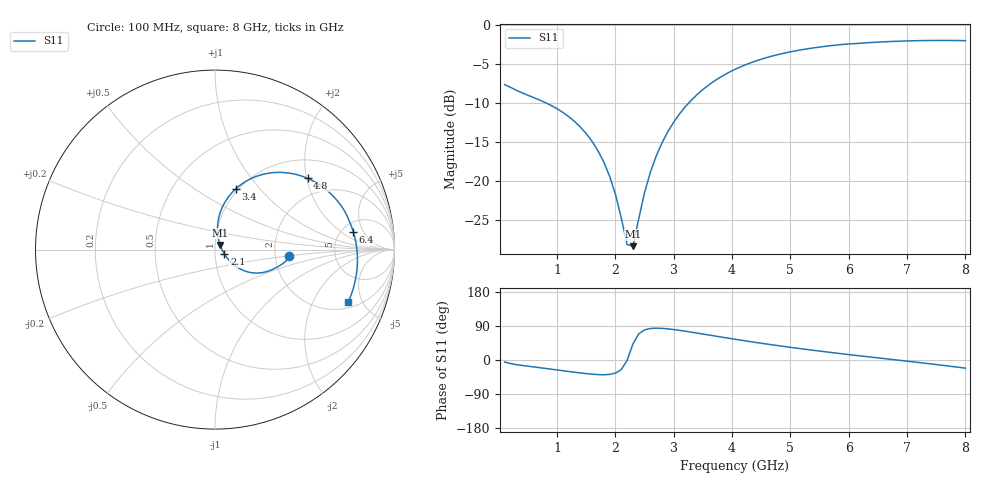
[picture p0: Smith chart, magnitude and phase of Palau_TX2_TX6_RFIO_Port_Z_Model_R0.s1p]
! Created Wed Jul  8 18:09:28 2020
! Palau TX2/TX6 RFIO Port Impedance Model.
! Revision		: R0.
! Impedance Mode 	: Balanced Differential-Mode.
! Impedance Format 	: Series Equivalent Differential Impedance (SEDZ).
# hz S ma R 50
! 1 Port Network Data from SP1.SP block
! freq  magS11  angS11
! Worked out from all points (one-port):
!   80 points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, 100 MHz to 8 GHz, reference 50 ohm
!   lowest |S11| = -28.4 dB at 2.3 GHz (marker M1), VSWR 1.08, Z = 52.8 + j2.7 ohm
!   |S11| at or under -10 dB: 817.6 MHz to 3.254 GHz (2.437 GHz wide, 120 % of centre)
!   S11 on the Smith chart (normalised r, x): 100 MHz: 2.40, -0.22; 2.1 GHz: 1.11, -0.06; 3.4 GHz: 0.97, +0.76; 4.8 GHz: 1.47, +2.02; 6.4 GHz: 6.34, +3.17; 8 GHz: 2.39, -3.85
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1e8  0.4161 -5.3
4e8  0.3683 -14.4
1.1e9  0.2756 -28.3
1.4e9  0.2217 -34.2
1.7e9  0.1563 -38.5
1.9e9  0.1073 -38.0
2e9  0.08201 -34.7
2.1e9  0.05775 -25.4
2.2e9  0.03896 -1.0
2.3e9  0.03802 42.1
2.5e9  0.08421 79.5
2.6e9  0.114 83.1
2.7e9  0.1448 84.0
2.8e9  0.1762 83.4
2.9e9  0.2076 82.1
3.1e9  0.2699 78.2
3.4e9  0.359 71.1
3.8e9  0.4647 61.0
4.1e9  0.5322 53.5
4.4e9  0.5894 46.5
4.8e9  0.6509 37.6
5.1e9  0.6875 31.4
5.6e9  0.734 21.7
6.1e9  0.7637 12.5
6.4e9  0.7769 7.3
7.1e9  0.7964 -4.8
7.6e9  0.8003 -13.8
8e9  0.798 -21.5
